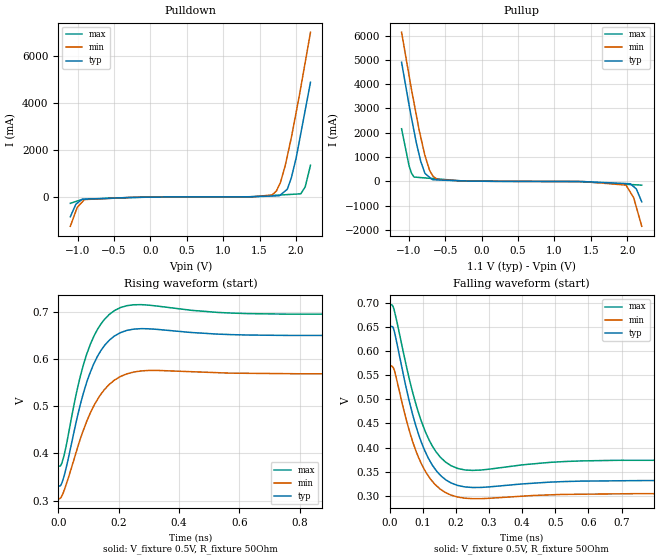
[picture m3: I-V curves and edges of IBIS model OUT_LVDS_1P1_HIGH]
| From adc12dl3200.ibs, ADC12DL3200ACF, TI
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|   OUT_LVDS_1P1_HIGH
[Model]   OUT_LVDS_1P1_HIGH
Model_type   Output
Polarity   Non-Inverting
Vmeas = 0.5
Vref = 0.5
Cref = 2pF
Rref = 50
|   typ   min   max
C_comp   1.769E-12   1.713E-12   1.772E-12
[Voltage Range]   1.1   1.05   1.15
[Temperature Range]   90   150   -55
[Pullup Reference]   1.1   1.05   1.15
[Pulldown Reference]   0   -0   0
[Power Clamp Reference]   1.1   1.05   1.15
[GND Clamp Reference]   0   0   0
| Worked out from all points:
|   slope of the pulldown table from 0 to 0.165 V, typ, clamps not added: 32.9 ohm
|   slope of the pullup table from 0 to 0.165 V, typ, clamps not added: 43.2 ohm
|   falling waveform, V_fixture 0.5V, R_fixture 50Ohm: 20-80 % time 74.4ps typ, 73ps min, 73.7ps max; typ from 0.651 V to 0.331 V
|   rising waveform, V_fixture 0.5V, R_fixture 50Ohm: 20-80 % time 80ps typ, 93.6ps min, 73.2ps max; typ from 0.331 V to 0.651 V
[Pulldown]
|   Voltage   I(typ)   I(min)   I(max)
-1.1V     -842.3mA   -1.25A     -268.7mA
-1.005V   -259mA     -439mA     -171.9mA
-905.9mV  -91.81mA   -108.1mA   -95.26mA
1.674V    43.25mA    93.94mA    66.58mA
1.732V    50.1mA     259.8mA    76.9mA
1.791V    102.1mA    662.3mA    87.49mA
1.878V    323.9mA    1.706A     103.1mA
1.936V    808.4mA    2.523A     113.4mA
2.003V    1.662A     3.614A     125.4mA
2.067V    2.719A     4.688A     140.3mA
2.127V    3.701A     5.744A     431.6mA
2.2V      4.9A       7.032A     1.356A
[Pullup]
|   Voltage   I(typ)   I(min)   I(max)
-1.1V     4.9A       6.135A     2.163A
-998.2mV  3.158A     4.37A      652.9mA
-963.9mV  2.609A     3.778A     333.8mA
-836.2mV  815.5mA    1.812A     153.2mA
-776.9mV  318.2mA    1.04A      138.9mA
-717.6mV  171.2mA    472.7mA    124.7mA
-665.5mV  63.62mA    198.4mA    112.2mA
-265mV    15.4mA     14.38mA    17.07mA
1.981V    -91.6mA    -155.7mA   -120.9mA
2.089V    -219.3mA   -672mA     -139.3mA
2.125V    -312.7mA   -1.058A    -145.5mA
2.2V      -843.4mA   -1.852A    -158.2mA
[Ramp]
R_load = 50
|   typ   min   max
dV/dt_r   0.191576/7.99318e-11   0.158971/9.35796e-11   0.193146/7.31501e-11
dV/dt_f   0.191576/7.44701e-11   0.15897/7.31149e-11   0.193138/7.3716e-11
[Falling Waveform]
V_fixture = 0.5V
V_fixture_min = 0.45V
V_fixture_max = 0.55V
R_fixture = 50Ohm
C_fixture = 0F
|   Time   V(typ)   V(min)   V(max)
0s        650.6mV    569.1mV    695.6mV
12.57ps   644.9mV    563.3mV    687.6mV
68.76ps   470.5mV    414.2mV    516.6mV
89.17ps   423.7mV    376.7mV    468.3mV
116.1ps   378.9mV    341.9mV    420.2mV
140.6ps   352.4mV    321.5mV    390.7mV
168.6ps   333.7mV    306.9mV    370mV
227.5ps   318.4mV    295.1mV    353.6mV
690.5ps   331.2mV    304.1mV    373.6mV
5ns       331.3mV    304.1mV    373.7mV
[Rising Waveform]
V_fixture = 0.5V
V_fixture_min = 0.45V
V_fixture_max = 0.55V
R_fixture = 50Ohm
C_fixture = 0F
|   Time   V(typ)   V(min)   V(max)
0s        331.3mV    304.1mV    373.7mV
7.76ps    332.3mV    305.6mV    374.2mV
15.77ps   345.1mV    315.9mV    388mV
72.72ps   503.2mV    430.6mV    563.4mV
93.6ps    550mV      467.2mV    610mV
119.2ps   592.5mV    502.8mV    650.8mV
170.2ps   641.2mV    547.2mV    695.7mV
250.4ps   664mV      572.9mV    715.7mV
759.3ps   650.6mV    569.4mV    695.8mV
5ns       650.6mV    569.1mV    695.6mV
